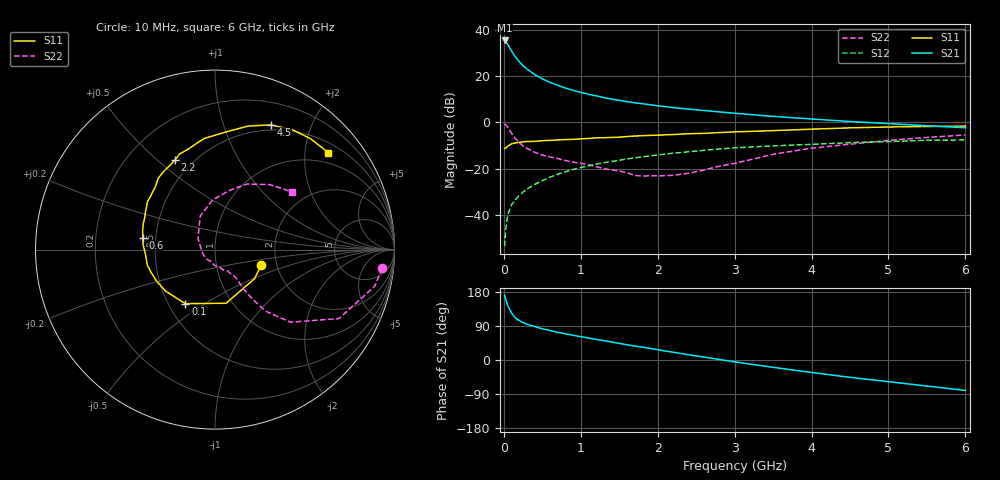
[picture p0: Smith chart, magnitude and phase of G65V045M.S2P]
! SIEMENS Small Signal Semiconductors
! BFG193
! Si NPN RF Bipolar Junction Transistor in SOT223
! VCE = 5 V  IC = 45 mA
! Common Emitter S-Parameters:  August  1996
# GHz  S  MA  R  50
!  f  S11  S21  S12  S22
! GHz  MAG  ANG  MAG  ANG  MAG  ANG  MAG  ANG
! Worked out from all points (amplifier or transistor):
!   36 points, 10 MHz to 6 GHz, reference 50 ohm
!   highest |S21| = 35.4 dB at 10 MHz (marker M1)
!   |S21| within 3 dB of that: start of sweep to 73.44 MHz
!   unconditionally stable (mu >= 1): 457.9 MHz to 2.357 GHz
!   at 250 MHz: K = 0.89, MSG = 27.3 dB, |S12| = -30.1 dB
!   at 1.4 GHz: K = 1.04, MAG = 12.2 dB, |S12| = -16.9 dB
!   at 6 GHz: K = 0.89, MSG = 2.6 dB, |S12| = -7.6 dB
!   S11 on the Smith chart (normalised r, x): 10 MHz: 1.66, -0.31; 100 MHz: 0.61, -0.42; 600 MHz: 0.42, +0.07; 2.2 GHz: 0.40, +0.57; 4.5 GHz: 0.44, +1.45; 6 GHz: 0.72, +2.52
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0.01  0.2723 -18.7  59.12 171.2  0.0021 91.5  0.9378 -6.4
0.02  0.2737 -36.4  57.33 163.9  0.0042 76.1  0.9119 -13.0
0.05  0.305 -78.4  48.85 143.6  0.0099 73.9  0.7902 -29.1
0.1  0.3436 -118.7  35.13 123.8  0.0164 67.3  0.5831 -43.9
0.15  0.3593 -139.9  25.98 111.2  0.0213 65.0  0.4454 -50.5
0.2  0.3699 -151.4  20.55 104.2  0.0262 67.4  0.3665 -52.3
0.25  0.3779 -160.4  16.81 98.6  0.0311 67.1  0.3083 -53.5
0.3  0.387 -167.0  14.23 94.4  0.0359 69.0  0.2745 -54.0
0.4  0.3879 -176.0  10.86 88.3  0.0454 68.4  0.2255 -53.7
0.5  0.4016 176.0  8.727 82.4  0.055 67.8  0.1966 -53.4
0.6  0.4076 170.5  7.338 77.8  0.0654 66.8  0.1797 -54.4
0.7  0.4167 165.5  6.325 73.2  0.0754 65.6  0.1646 -56.3
0.8  0.4242 160.8  5.528 69.1  0.0853 64.0  0.1493 -58.1
1.1  0.4491 148.3  4.059 58.1  0.1148 59.0  0.1212 -68.1
1.3  0.4645 141.5  3.45 50.9  0.1341 55.0  0.0998 -75.9
1.6  0.4938 131.1  2.809 40.2  0.1616 48.1  0.0813 -96.5
2.2  0.5456 114.3  2.088 20.6  0.2153 34.7  0.0715 -159.4
2.8  0.601 99.7  1.684 1.4  0.2657 20.9  0.1128 146.8
3.5  0.6628 83.7  1.349 -19.3  0.3106 3.7  0.2038 113.9
4.5  0.7612 65.9  1.044 -45.7  0.365 -16.3  0.3378 76.7
5.5  0.8159 49.1  0.846 -68.7  0.411 -39.5  0.4733 49.9
6  0.8307 40.6  0.765 -80.3  0.4167 -53.0  0.5346 37.1
